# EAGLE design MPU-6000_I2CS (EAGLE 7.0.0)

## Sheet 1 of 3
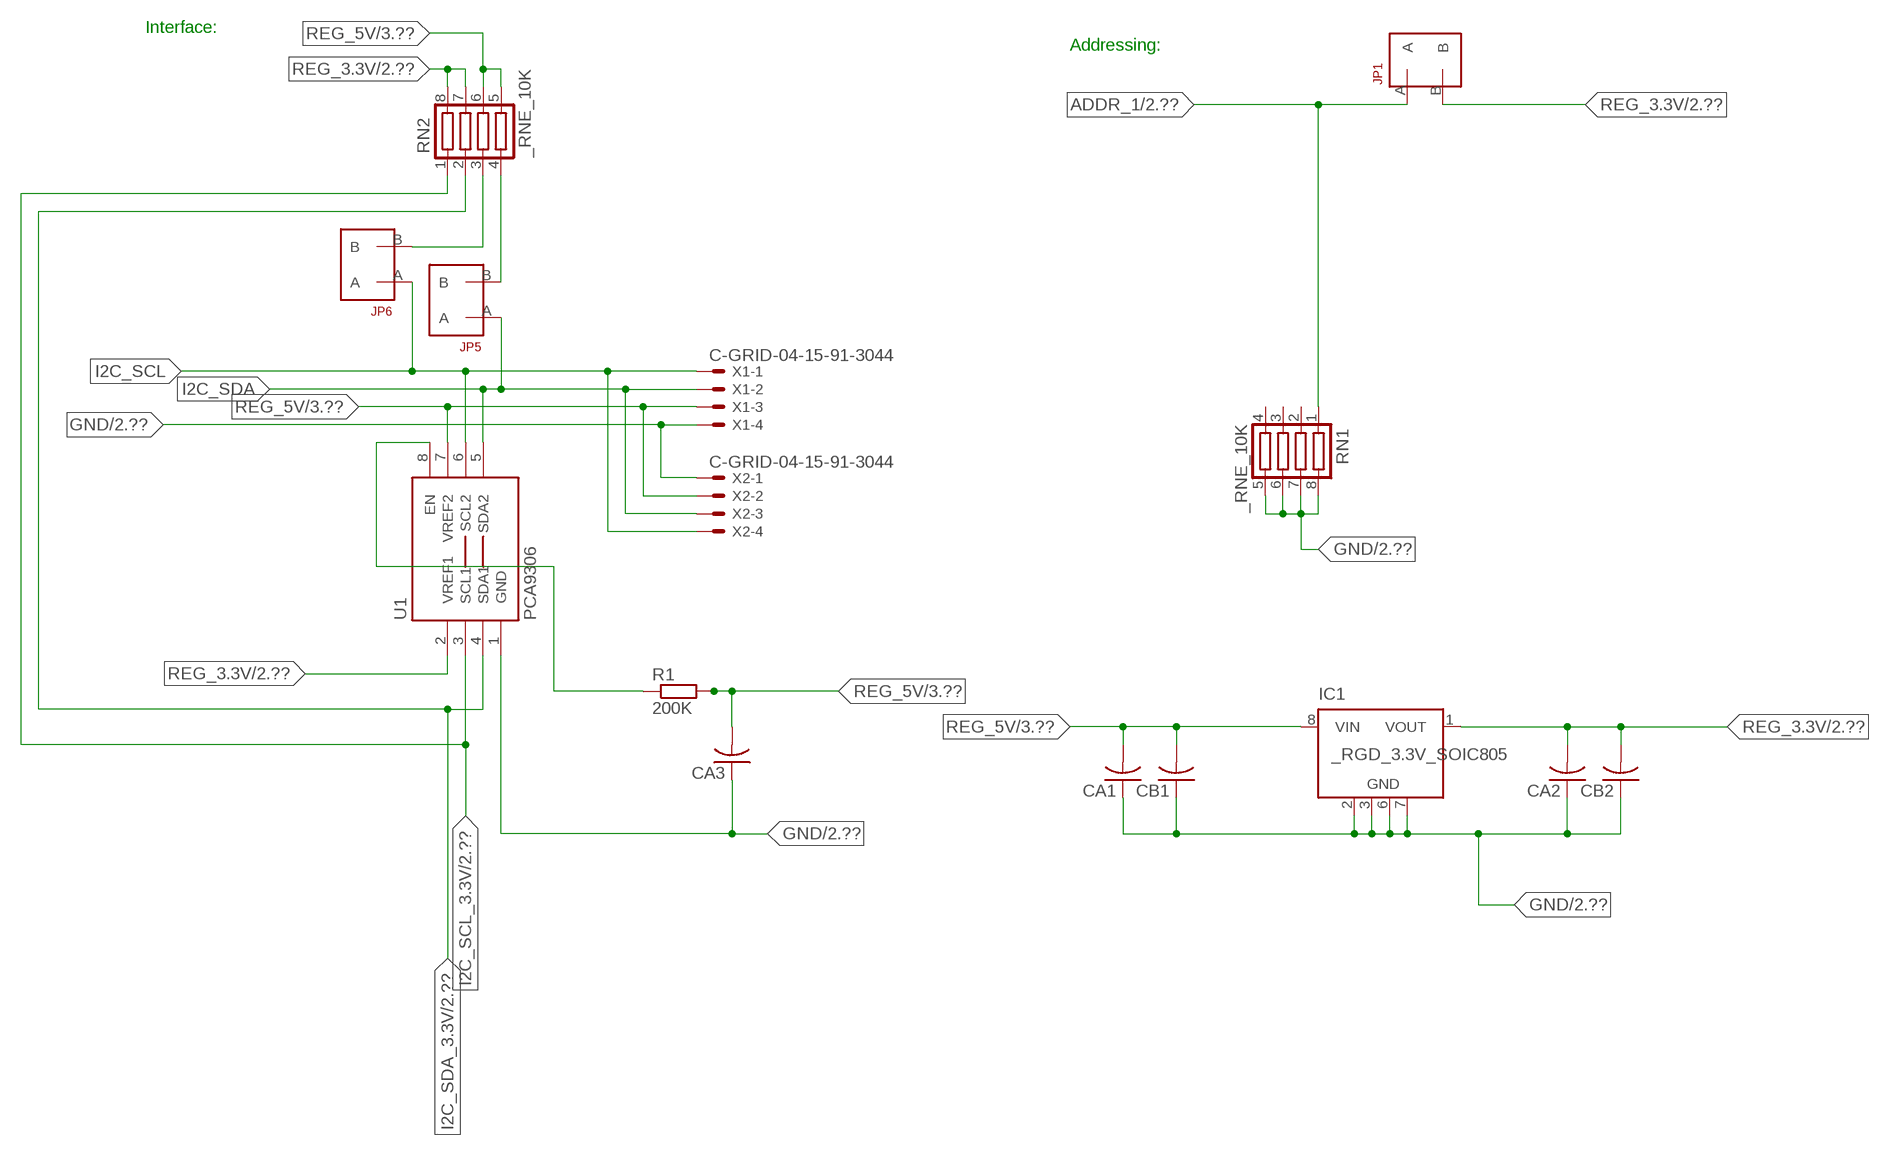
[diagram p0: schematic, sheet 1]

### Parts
CA1  CC1206KRX7R9BB104  [.1UF]
CA2  CC1206KRX7R9BB104  [.1UF]
CA3  CC1206KRX7R9BB104  [.1UF]
CB1  TMK316F106ZL-TC1206K  [TMK316F106ZL-T]
CB2  TMK316F106ZL-TC1206K  [TMK316F106ZL-T]
IC1  _RGD_3.3V_SOIC805  [_RGC_3.3V_SOIC8]
JP1  JUMPER_1X2_2MM  [JUMPER_1X2_2MM]
JP5  JUMPER_1X2_2MM  [JUMPER_1X2_2MM]
JP6  JUMPER_1X2_2MM  [JUMPER_1X2_2MM]
R1  200K  RESISTOR_SMT-0603  [R603]
RN1  _RNE_10K  [RNE]
RN2  _RNE_10K  [RNE]
U1  PCA9306  PCA9306_NCD  [PSOP-8]
X1  C-GRID-04-15-91-3044  [15-91-04]
X2  C-GRID-04-15-91-3044  [15-91-04]

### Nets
ADDR_1: JP1.A RN1.1 ; also sheet 2
GND: CA1.1 CA2.1 CA3.1 CB1.1 CB2.1 IC1.2(GND) IC1.3(GND) IC1.6(GND) IC1.7(GND) RN1.5 RN1.6 RN1.7 RN1.8 U1.1(GND) X1.4 X2.1 ; also sheet 2,3
I2C_SCL: JP6.A U1.6(SCL2) X1.1 X2.4
I2C_SCL_3.3V: RN2.1 U1.3(SCL1) ; also sheet 2
I2C_SDA: JP5.A U1.5(SDA2) X1.2 X2.3
I2C_SDA_3.3V: RN2.2 U1.4(SDA1) ; also sheet 2
N$1: JP6.B RN2.3
N$2: JP5.B RN2.4
N$3: R1.1 U1.8(EN)
REG_3.3V: CA2.2 CB2.2 IC1.1(VOUT) JP1.B RN2.7 RN2.8 U1.2(VREF1) ; also sheet 2
REG_5V: CA1.2 CA3.2 CB1.2 IC1.8(VIN) R1.2 RN2.5 RN2.6 U1.7(VREF2) X1.3 X2.2 ; also sheet 3
Unconnected: IC1.4(NC) IC1.5(NC) RN1.2 RN1.3 RN1.4

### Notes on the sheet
- Interface:
- Addressing:

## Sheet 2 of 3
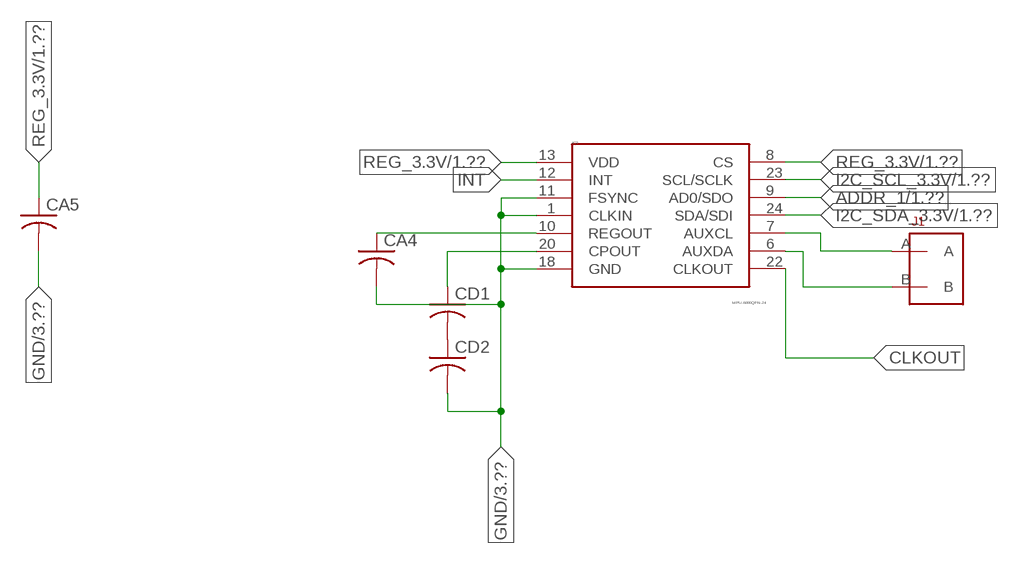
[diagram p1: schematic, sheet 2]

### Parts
CA4  CC1206KRX7R9BB104  [.1UF]
CA5  CC1206KRX7R9BB104  [.1UF]
CD1  _CD_10NF_50VC1206K  [_CD_10NF_50V]
CD2  _CD_10NF_50VC1206K  [_CD_10NF_50V]
IC2  MPU-6000QFN-24  [QFN-24-TESTING]
J1  JUMPER_1X2_2MM  [JUMPER_1X2_2MM]

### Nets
ADDR_1: IC2.9(AD0/SDO) ; also sheet 1
CLKOUT: IC2.22(CLKOUT)
GND: CA4.2 CA5.2 CD2.2 IC2.1(CLKIN) IC2.11(FSYNC) IC2.18(GND) ; also sheet 1,3
I2C_SCL_3.3V: IC2.23(SCL/SCLK) ; also sheet 1
I2C_SDA_3.3V: IC2.24(SDA/SDI) ; also sheet 1
INT: IC2.12(INT)
N$18: CA4.1 IC2.10(REGOUT)
N$19: CD1.1 IC2.20(CPOUT)
N$25: CD1.2 CD2.1
N$53: IC2.7(AUXCL) J1.A
N$54: IC2.6(AUXDA) J1.B
REG_3.3V: CA5.1 IC2.8(CS) IC2.13(VDD) ; also sheet 1

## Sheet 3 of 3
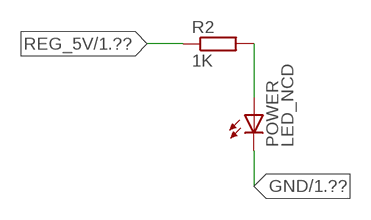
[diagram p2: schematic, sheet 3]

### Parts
POWER  LED_NCD  [CHIPLED_0603]
R2  1K  RESISTOR_SMT-0402  [R402]

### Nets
GND: POWER.C ; also sheet 1,2
N$4: POWER.A R2.2
REG_5V: R2.1 ; also sheet 1

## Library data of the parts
CA1-CA3 = NCD_ULTIMATE_LIBRARY:CC1206KRX7R9BB104: Capacitor CA .1uF 50V SMT C1206K CC1206KRX7R9BB104
CA4 CA5 = NCD_ULTIMATE_LIBRARY (2):CC1206KRX7R9BB104: Capacitor CA .1uF 50V SMT C1206K CC1206KRX7R9BB104
CB1 CB2 = NCD_ULTIMATE_LIBRARY:TMK316F106ZL-T: Capacitor CB 10uF SMT 1206 TMK316F106ZL-T
CD1 CD2 = NCD_ULTIMATE_LIBRARY (2):_CD_10NF_50V: Capacitor 10nF SMT
IC1 = NCD_ULTIMATE_LIBRARY:_RGD_3.3V_SOIC8: Regulator Linear 3.3V Chip Positive VOLTAGE REGULATOR Digikey 497-1199-2-ND/L78L33ACD13TR
IC2 = NCD_ULTIMATE_KAMNA:MPU-6000: MPU-6000 - I2C address is 0x68 with AD0 low and 0x69 with AD0 high.
J1 JP1 JP5 JP6 = NCD_ULTIMATE_CONNECTORS:JUMPER_1X2_2MM
POWER = NCD_ULTIMATE_LIBRARY:LED_NCD: LED Digikey 754-1132-2-ND/APT2012SRCPRV
R1 R2 = NCD_ULTIMATE_LIBRARY:RESISTOR_SMT: NCD Resistor
RN1 RN2 = NCD_ULTIMATE_LIBRARY:_RNE_10K: Resistor Array RNE SMT 10K x 4 Single Resistor Source: http://www.ctscorp.com/components/Datasheets/CTSChipArrayDs.pdf Digikey 742C083103JPTR-ND/742C083103JP; OC_FARNELL: unknown; OC_NEWARK: unknown
U1 = NCD_ULTIMATE_LIBRARY:PCA9306_NCD: NCD Bidirectional I2C level shifter. NOT compatible with all available part number pinout schemes- DOUBLE CHECK!!!; PROD_ID: IC-10023
X1 X2 = NCD_ULTIMATE_CONNECTORS:C-GRID-04: CONNECTOR 4-Pos I2C wire to board 2.54 mm (0.100") pitch header Digikey WM1342-ND/0015912045; OC_FARNELL: unknown; OC_NEWARK: unknown

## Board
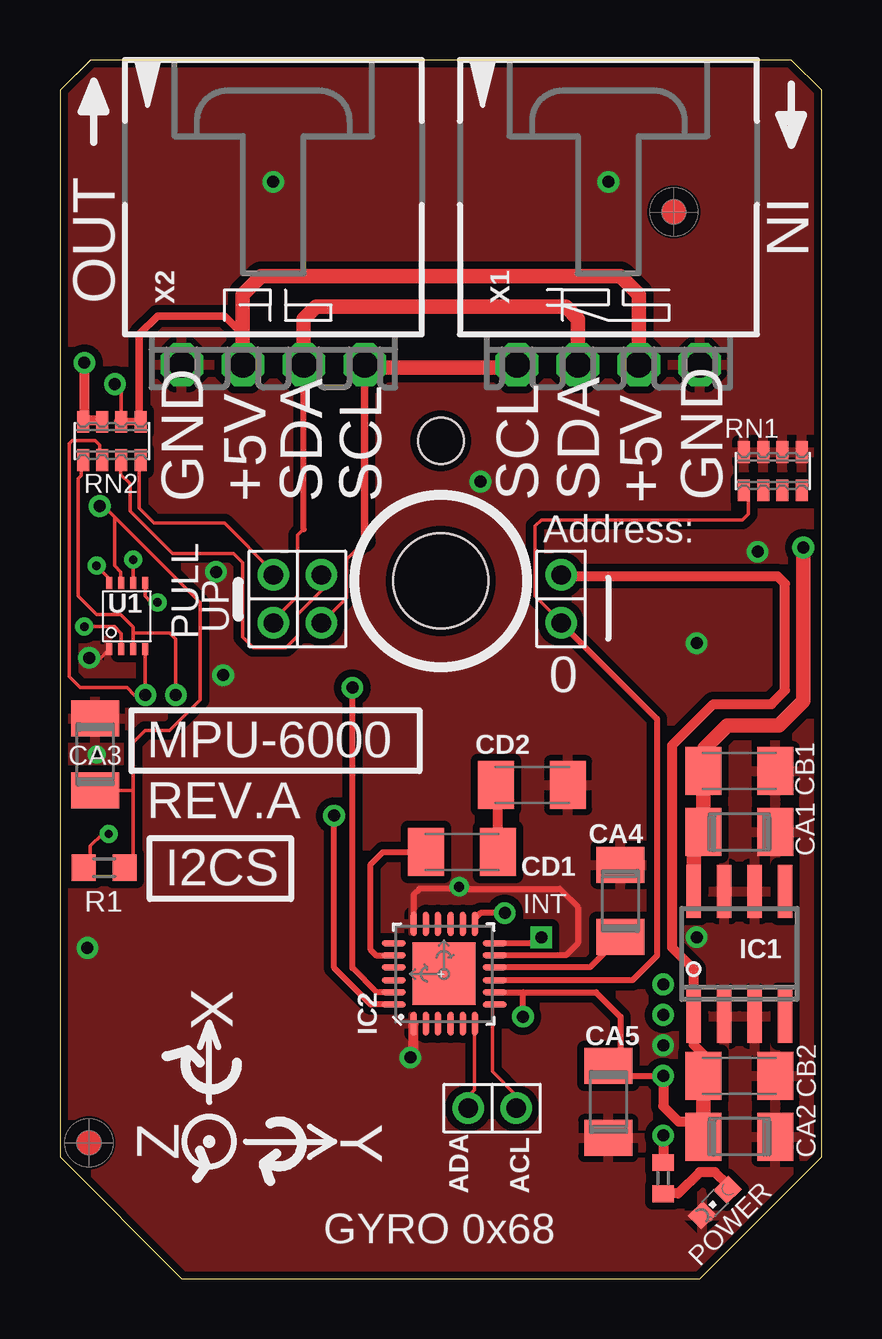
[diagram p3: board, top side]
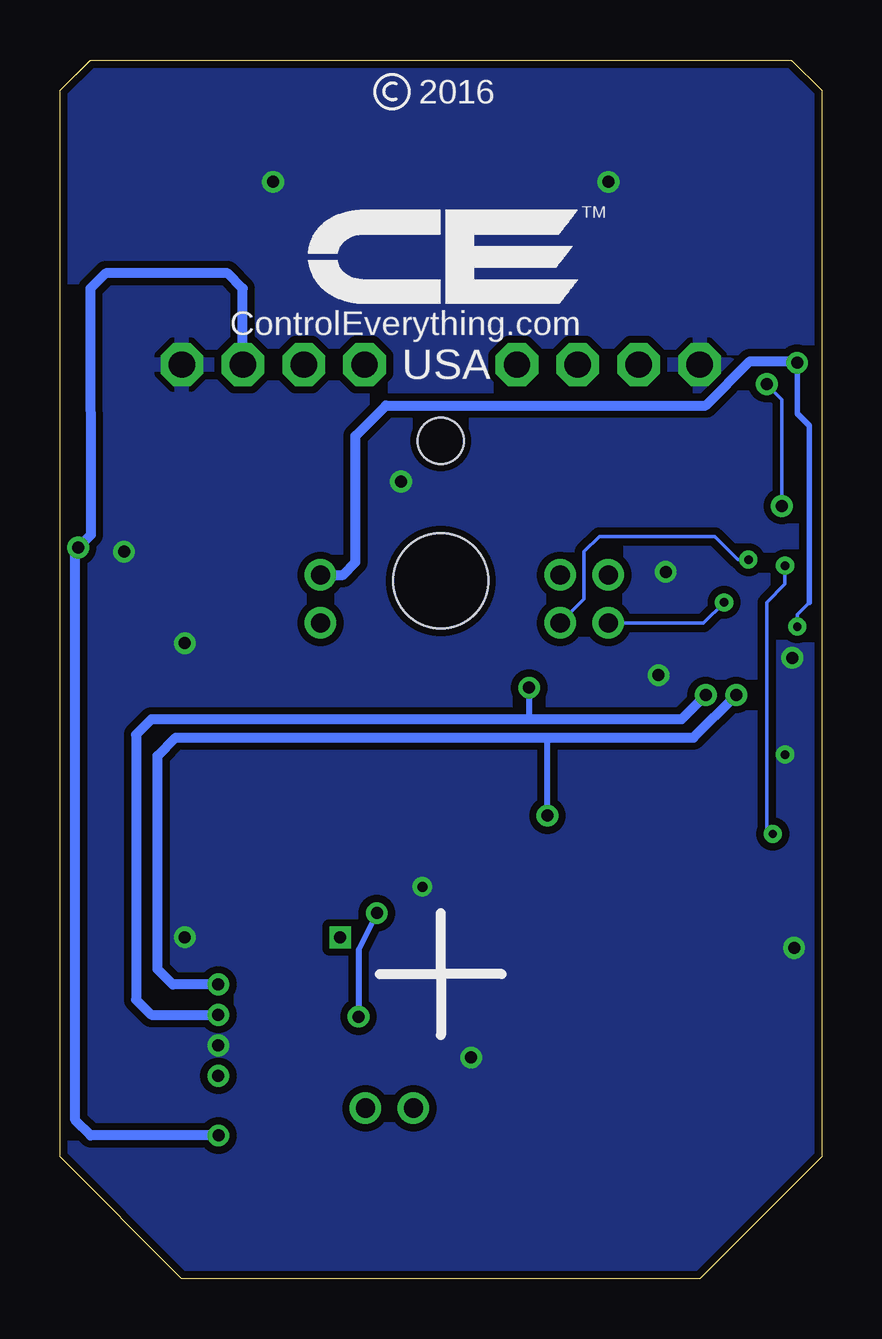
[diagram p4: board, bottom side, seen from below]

Size 31.75 x 50.8 mm. Coordinates in mm from the lower left corner, seen from the top.
Outline: 32 segments
Copper layers (1*16): Top 0.035mm / dielectric 1.5mm / Bottom 0.035mm
Design rules "default": minimum track width 5mil, minimum drill 24mil, track to track 5mil, track to pad 5mil, pad to pad 5mil, via to via 5mil, smd to smd 5mil, copper to edge 10mil, drill to drill 8mil, minimum pad ring 10mil, minimum via ring 8mil, stop-mask expansion 2mil, vias tented up to drill 0mil, thermal gap 10mil
Holes 3.96 mm at 15.88,29.08
Holes 1.91 mm at 15.88,34.93

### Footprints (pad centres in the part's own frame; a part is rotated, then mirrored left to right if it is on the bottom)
.1UF = smd 1.5 x 2: 1 -1.5,0; 2 1.5,0
TMK316F106ZL-T = smd 1.5 x 2: 1 -1.5,0; 2 1.5,0
_CD_10NF_50V = smd 1.5 x 2: 1 -1.5,0; 2 1.5,0
_RGC_3.3V_SOIC8 = smd 0.6 x 2.2: 1 -1.905,-2.6; 2 -0.635,-2.6; 3 0.635,-2.6; 4 1.905,-2.6; 5 1.905,2.6; 6 0.635,2.6; 7 -0.635,2.6; 8 -1.905,2.6
QFN-24-TESTING = smd 1.016 x 0.254: 1 -2.066,1.257; 2 -2.066,0.75; 3 -2.066,0.247; 4 -2.066,-0.287; 5 -2.066,-0.792; 6 -2.066,-1.297; 13 2.086,-1.297; 14 2.086,-0.792; 15 2.086,-0.287; 16 2.086,0.247; 17 2.086,0.75; 18 2.086,1.257 | smd 0.254 x 1.016: 7 -1.267,-2.122; 8 -0.762,-2.122; 9 -0.258,-2.122; 10 0.278,-2.122; 11 0.78,-2.122; 12 1.287,-2.122; 19 1.287,2.082; 20 0.78,2.082; 21 0.278,2.082; 22 -0.258,2.082; 23 -0.762,2.082; 24 -1.267,2.082 | smd 2.616 x 2.616: P$1 0.02,-0.01
JUMPER_1X2_2MM = drill 0.8: A 0,2; B 0,0
CHIPLED_0603 = smd 0.8 x 0.876: A 0,-0.75; C 0,0.75
R603 = smd 1 x 1.1: 1 -0.85,0; 2 0.85,0
R402 = smd 0.7 x 0.9: 1 -0.65,0; 2 0.65,0
RNE = smd 0.5 x 0.9: 1 -1.2,-0.8; 2 -0.4,-0.8; 3 0.4,-0.8; 4 1.2,-0.8; 5 1.2,0.8; 6 0.4,0.8; 7 -0.4,0.8; 8 -1.2,0.8
PSOP-8 = smd 0.25 x 0.5: 1 -0.73,-1.37; 2 -0.23,-1.37; 3 0.27,-1.37; 4 0.77,-1.37; 5 0.77,1.38; 6 0.27,1.38; 7 -0.23,1.38; 8 -0.73,1.38
15-91-04 = drill 1.1 pad 1.778 octagon: 1 -3.81,-7.62; 2 -1.27,-7.62; 3 1.27,-7.62; 4 3.81,-7.62

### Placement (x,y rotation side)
CA1  28.32,18.62 180 top
CA2  28.32,5.92 180 top
CA3  1.46,21.86 270 top
CA4  23.37,15.75 90 top
CA5  22.86,7.37 270 top
CB1  28.32,21.16 180 top
CB2  28.32,8.46 180 top
CD1  16.76,17.78 0 top
CD2  19.68,20.57 0 top
IC1  28.32,13.54 0 top
IC2  16,12.7 90 top
J1  17.02,7.11 270 top
JP1  20.89,29.34 180 top
JP5  8.89,29.34 180 top
JP6  10.9,29.34 180 top
POWER  27.3,3.18 135 top
R1  1.84,17.13 0 top
R2  25.15,4.19 270 top
RN1  29.72,33.66 0 top
RN2  2.16,34.93 0 top
U1  2.79,27.61 0 top
U$5  [VISION_REF10]  1.21,5.66 90 top
U$28  [VISION_REF10]  25.59,44.46 90 top
X1  22.86,45.72 0 top
X2  8.89,45.72 0 top

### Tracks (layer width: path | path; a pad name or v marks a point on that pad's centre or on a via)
ADDR_1
  Top 0.152: JP1.A 20.89,27.37 19.81,28.45 19.81,31.37 20.07,31.62 28.45,31.62 28.7,31.88 28.7,32.78 RN1.1
  Top 0.254: JP1.A 24.89,23.34 24.89,13.46 23.87,12.44 IC2.9
GND  (via drill 0.35, 0.41, 0.5)
  Top 0.152: CA3.1 1.52,23.42 1.52,23.62 | U1.1 1.7,25.88 v1.22,25.88
  Top 0.254: IC2.18 14.74,16.02 14.99,16.26 16.56,16.26 v16.64,16.33 16.72,16.26 20.83,16.26 21.59,15.49 21.59,13.97 21.1,13.48 IC2.11
  Top 0.406: v14.61,9.22 14.74,9.36 IC2.1
  other vias: 8.89,45.72 22.86,45.72 25.15,9.73 6.8,25.16 17.53,33.22 26.55,14.24 1.15,13.79 6.5,29.46 1.52,21.84 26.55,26.49 29.09,30.3
  pour Top (isolate 0.305): -1.27,0 -1.27,50.8 33.02,50.8 33.02,0
  pour Bottom (isolate 0.305): -5.08,0 -5.08,50.8 35.56,50.8 35.56,0
I2C_SCL  (via drill 0.35)
  Top 0.152: 12.7,30.73 11.94,29.97 11.94,28.38 JP6.A | v3.05,29.97 3.06,29.96 U1.6
  Top 0.305: 12.7,30.73 X2.4
  Top 0.406: X2.4 12.7,37.97 | 19.05,37.97 X1.1
  Top 0.61: 12.7,37.97 19.05,37.97
  Bottom 0.152: JP6.A 9.91,28.33 9.91,30.3 9.27,30.94 4.45,30.94 3.48,29.97 v3.05,29.97
I2C_SCL_3.3V  (via drill 0.5)
  Top 0.152: RN2.1 0.89,34.07 0.89,33.48 0.77,33.35 0.77,29.1 0.76,29.09 0.76,28.45 1.52,27.69 2.54,27.69 3.06,27.17 3.06,26.92 | 3.06,26.92 U1.3 | v4.83,24.33 v4.83,24.34 4.83,26.67 4.57,26.92 3.06,26.92
  Top 0.254: IC2.23 | IC2.23 13.21,11.94 12.19,12.95 v12.19,24.64
  Bottom 0.254: v12.19,24.64 12.19,23.32
  Bottom 0.406: v4.83,24.33 5.84,23.32 12.19,23.32 27.94,23.32 28.58,22.68 28.58,11.63 27.94,11 v25.15,11
I2C_SDA  (via drill 0.35)
  Top 0.152: JP5.A 8.89,27.44 9.91,28.45 9.91,30.99 10.16,31.24 | U1.5 3.56,28.45 3.81,28.19 v4.06,28.19
  Top 0.254: 10.16,31.24 10.16,31.25 X2.3
  Top 0.61: X2.3 10.16,40.01 10.67,40.51 21.09,40.51 21.59,40.01 X1.2
  Bottom 0.152: v4.06,28.19 4.92,27.34 JP5.A
I2C_SDA_3.3V  (via drill 0.5)
  Top 0.152: RN2.2 1.65,34.14 1.65,34.75 1.46,34.94 0.51,34.94 0.38,34.81 0.38,26.37 0.38,26.36 0.38,25.1 0.84,24.64 2.79,24.64 3.1,24.33 v3.56,24.33 v3.56,24.34 U1.4
  Top 0.254: IC2.24 12.95,11.43 11.43,12.95 v11.43,19.3
  Bottom 0.254: v11.43,19.3 11.43,22.56
  Bottom 0.406: v25.15,12.27 27.05,12.27 27.69,12.9 27.69,21.79 26.93,22.56 11.43,22.56 5.34,22.56 v3.56,24.33
INT  (via drill 0.5)
  Top 0.254: IC2.12 19.83,13.99 v20.07,14.22
N$1
  Top 0.152: JP6.B 10.92,29.31 10.92,28.7 9.91,27.69 9.91,26.8 9.42,26.31 8.06,26.31 7.62,26.75 7.62,29.84 7.24,30.23 4.7,30.23 2.92,32 2.92,33.15 2.54,33.53 2.54,34.1 RN2.3
  Top 0.305: 2.54,34.02 RN2.3
N$2
  Top 0.152: JP5.B 8.89,29.46 6.86,31.5 3.94,31.5 3.3,32.13 3.3,34.07 RN2.4
  Top 0.305: 3.37,33.88 RN2.4
N$3  (via drill 0.35)
  Top 0.152: R1.1 1.27,17.41 1.27,18.03 1.78,18.54 v2.03,18.54 | v1.52,29.72 2.06,29.18 U1.8
  Bottom 0.152: v2.03,18.54 2.29,18.8 2.29,28.19 1.52,28.96 v1.52,29.72
N$4
  Top 0.406: POWER.A 27.84,3.92 27.3,4.45 26.67,4.45 25.78,3.56 25.16,3.56 R2.2
N$18
  Top 0.254: CA4.1 22.1,12.98 IC2.10
N$19
  Top 0.254: IC2.20 13.9,13.46 13.21,13.46 12.95,13.72 12.95,17.27 13.46,17.78 CD1.1
N$25
  Top 0.406: CD1.2 18.26,20.5 CD2.1
N$53
  Top 0.152: IC2.7 18.03,11.34 18.03,8.64 19.02,7.65 J1.A
N$54
  Top 0.152: IC2.6 17.27,10.61 17.27,7.87 17.02,7.62 J1.B
REG_3.3V  (via drill 0.35, 0.5)
  Top 0.152: v1.02,27.18 2.29,27.18 2.56,26.9 U1.2
  Top 0.254: IC2.8 | IC2.8 19.3,11.94 | 19.3,11.94 22.35,11.94 23.37,10.92 23.37,8.89 23.34,8.87 CA5.1 23.27,8.46 v25.15,8.46 | v19.3,10.92 19.3,11.94 | v18.54,15.24 17.53,15.24 17.3,15.01 IC2.13
  Top 0.406: CB2.2 26.82,9.35 26.42,9.75 26.42,10.36 | v25.15,8.46 25.15,7.19 25.78,6.55 26.82,6.55 | IC1.1 26.42,12.9 25.53,13.79 25.53,22.24 27.24,23.95 29.66,23.95 30.23,24.52 30.23,28.97 29.91,29.29 20.95,29.29 JP1.B | 26.52,5.62 CA2.2 | v1.02,38.18 1.02,35.78 | 1.02,35.78 RN2.8 | 1.02,35.78 1.71,35.78 RN2.7
  Top 0.61: CB2.2 26.82,6.55 CA2.2 | 26.42,10.36 IC1.1
  Bottom 0.152: 0.51,28.19 1.02,27.69 v1.02,27.18
  Bottom 0.229: 0.51,28.19 0.51,35.56 1.02,36.07 v1.02,38.18
  Bottom 0.254: v18.54,15.24 19.3,13.72 v19.3,10.92
  Bottom 0.406: v1.02,38.18 1.08,38.24 2.99,38.24 4.83,36.4 18.16,36.4 19.43,35.13 19.43,29.87 19.94,29.34 JP1.B
REG_5V  (via drill 0.5)
  Top 0.152: RN2.6 2.56,37.01 v2.29,37.29 | R1.2 3.05,17.49 3.05,20.36 | 3.05,20.36 3.05,22.35 3.56,22.86 4.57,22.86 5.84,24.13 5.84,28.19 2.29,31.75 | CA3.2 3.05,20.36 | 2.29,31.75 1.83,32.21 v1.65,32.21 | U1.7 2.54,29.01 2.54,29.46 2.29,29.72 2.29,31.75
  Top 0.305: 7.62,39.37 7.5,39.37 | 2.42,35.74 RN2.6 RN2.5 3.31,35.8 3.31,39.37 4.07,40.13 6.86,40.13 7.62,39.37 | X2.2 7.62,39.37
  Top 0.406: v25.15,5.97 R2.1
  Top 0.61: X2.2 7.62,41.02 8.38,41.78 23.37,41.78 24.13,41.02 X1.3 | IC1.8 26.42,18.21 CA1.2 CB1.2 26.86,21.2 26.86,22.11 27.82,23.06 29.98,23.06 30.99,24.08 v30.99,30.48
  Bottom 0.152: v1.65,32.21 1.65,36.65 v2.29,37.29
  Bottom 0.406: X1.3 24.13,41.28 24.77,41.91 29.84,41.91 30.48,41.27 30.47,31 v30.99,30.48 31.11,30.36 31.11,6.6 30.48,5.97 v25.15,5.97

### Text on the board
tNames: IN | OUT | GND | +5V | SDA | SCL | SCL | SDA | +5V | GND | Address: | PULL | UP | 0 | MPU-6000 | REV.A | I2CS | INT | X | Y | Z | ADA | ACL | GYRO 0x68
bNames: 2016 | TM | ControlEverything.com | USA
